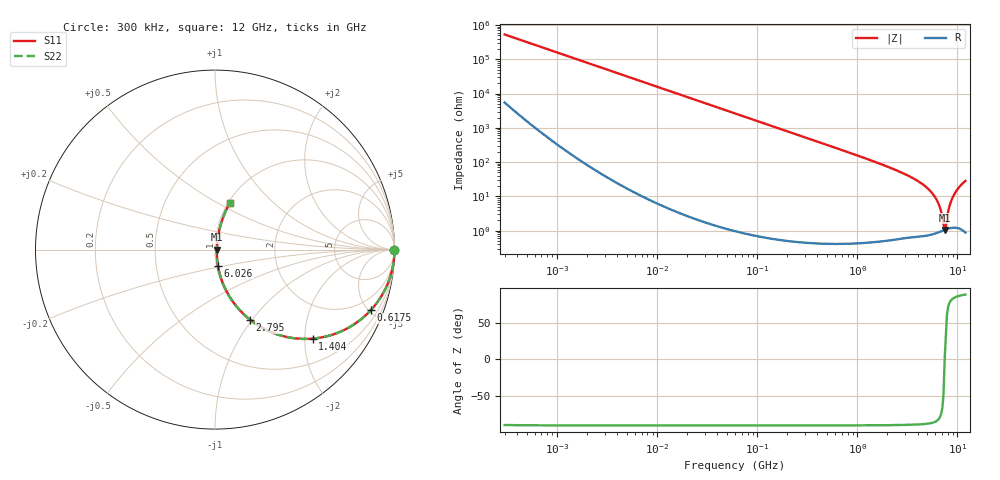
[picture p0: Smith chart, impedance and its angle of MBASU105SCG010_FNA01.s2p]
! MBASU105SCG010_FNA01  S-PARAMETER MODEL  ( Standard Model )
! Model Generated by TAIYO YUDEN Corporation (http://www.ty-top.com)
! Version 1.0
! TAIYO YUDEN Control No. 230609
! Copyright(c) 2023 TAIYO YUDEN CO.,LTD. All Rights Reserved.
! Product Description (link to TY-COMPAS)
! https://ds.yuden.co.jp/TYCOMPAS/or/detail?pn=MBASU105SCG010BFNA01&u=M
! Products Name : Multilayer Ceramic Capacitors
! Characteristics :
!  Capacitance : 1 [pF] , Rated Voltage : 50 [V] , TCC : CG / C0G
!  Case Size : 1.0 x 0.5 / 0.039 x 0.02 [mm/inch] , Thickness : 0.5 / 0.02 [mm/inch]
!  (Conditions: Temperature = 25 [degC] , DC Bias Voltage = 0 [V])
! External Node Assignments :
!  1  o---| |---o  2
! GND o---------o GND
! Frequency Range : 0.3MHz  -  12000MHz  [ 401 STEP ]
# MHZ S RI R 50
! Freq[MHz].  S11 Real  S11 Imag  S21 Real  S21 Imag  S12 Real  S12 Imag  S22 Real  S22 Imag
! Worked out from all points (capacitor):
!   401 points, 300 kHz to 12 GHz, reference 50 ohm
!   read as one part in series: C = 1 pF near 316.3 kHz
!   lowest |Z| = 1.05 ohm at 7.449 GHz (marker M1)
!   series resonance near 7.449 GHz, so ESL is about 460 pH
!   S11 on the Smith chart (normalised r, x): 300 kHz: open; 617.5 MHz: 1.01, -5.12; 1.404 GHz: 1.01, -2.19; 2.795 GHz: 1.01, -0.98; 6.026 GHz: 1.02, -0.18; 12 GHz: 1.02, +0.57
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0.3  1 -0.000188  1.98e-06 0.000188  1.98e-06 0.000188  1 -0.000188
1.769972  1 -0.00111  2.52e-06 0.00111  2.52e-06 0.00111  1 -0.00111
10.44266  1 -0.00656  4.56e-05 0.00656  4.56e-05 0.00656  1 -0.00656
60  0.9986 -0.0376  0.00143 0.0376  0.00143 0.0376  0.9986 -0.0376
159.8975  0.9899 -0.0995  0.0101 0.0995  0.0101 0.0995  0.9899 -0.0995
353.9943  0.9525 -0.2123  0.0475 0.2123  0.0475 0.2123  0.9525 -0.2123
617.4538  0.8672 -0.3386  0.1328 0.3386  0.1328 0.3386  0.8672 -0.3386
1403.667  0.5444 -0.4959  0.4556 0.4959  0.4556 0.4959  0.5444 -0.4959
2088.533  0.3314 -0.467  0.6686 0.467  0.6686 0.467  0.3314 -0.467
2795.104  0.196 -0.391  0.804 0.391  0.804 0.391  0.196 -0.391
4502.883  0.0538 -0.2108  0.9462 0.2108  0.9462 0.2108  0.0538 -0.2108
5278.635  0.029 -0.1447  0.971 0.1447  0.971 0.1447  0.029 -0.1447
6026.253  0.0163 -0.089  0.9837 0.089  0.9837 0.089  0.0163 -0.089
6524.734  0.0121 -0.0556  0.9879 0.0556  0.9879 0.0556  0.0121 -0.0556
7254.098  0.0102 -0.0111  0.9898 0.0111  0.9898 0.0111  0.0102 -0.0111
7448.838  0.0104 -9.79e-06  0.9896 9.79e-06  0.9896 9.79e-06  0.0104 -9.79e-06
7648.807  0.0108 0.00628  0.9892 -0.00628  0.9892 -0.00628  0.0108 0.00628
7854.144  0.0114 0.0195  0.9886 -0.0195  0.9886 -0.0195  0.0114 0.0195
8503.825  0.0155 0.0608  0.9845 -0.0608  0.9845 -0.0608  0.0155 0.0608
9207.246  0.0233 0.1052  0.9767 -0.1052  0.9767 -0.1052  0.0233 0.1052
10511.28  0.0462 0.1824  0.9538 -0.1824  0.9538 -0.1824  0.0462 0.1824
12000  0.0812 0.2581  0.9188 -0.2581  0.9188 -0.2581  0.0812 0.2581
